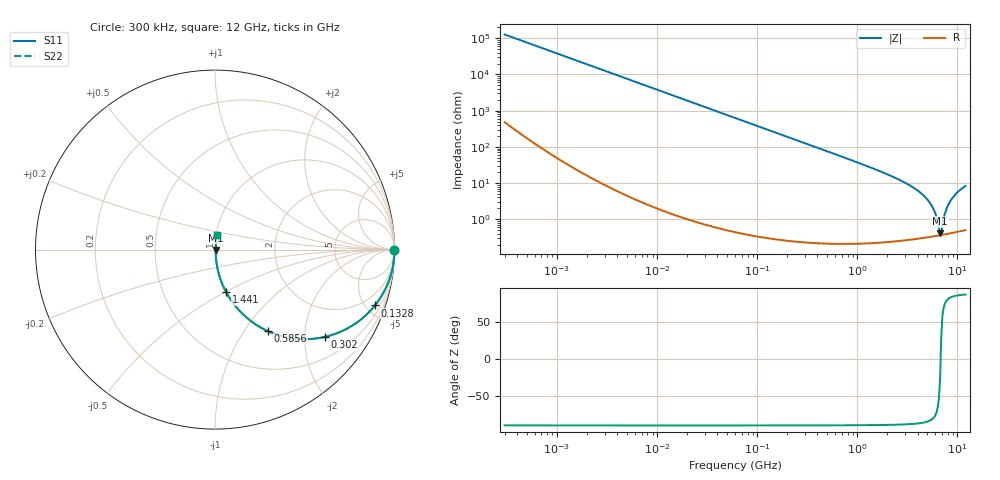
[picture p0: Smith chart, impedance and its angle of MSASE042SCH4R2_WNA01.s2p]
! MSASE042SCH4R2_WNA01  S-PARAMETER MODEL  ( General Type )
! Model Generated by TAIYO YUDEN Corporation (http://www.ty-top.com)
! Version 1.0
! TAIYO YUDEN Control No. 120810
! Copyright(c) 2012 TAIYO YUDEN CO.,LTD. All Rights Reserved.
! Product Description (link to TY-COMPAS)
! https://ds.yuden.co.jp/TYCOMPAS/or/detail?pn=MSASE042SCH4R2BWNA01&u=M
! Products Name : Multilayer Ceramic Capacitors
! Characteristics :
!  Capacitance : 4.2 pF , Rated Voltage : 16V , TCC : CH / C0H
!  Case Size : 0.4 x 0.2 / 0.016 x 0.008 [mm/inch] , Thickness : 0.2 / 0.008 [mm/inch]
!  (Conditions: Temperature = 25 degC , DC Bias Current/Voltage = 0A / 0V)
! External Node Assignments :
!  1  o---| |---o  2
! GND o---------o GND
! Frequency Range : 0.3MHz  -  12000MHz  [ 401 STEP ]
# MHz S RI R 50
! Freq[MHz].  S11 Real  S11 Imag  S21 Real  S21 Imag  S12 Real  S12 Imag  S22 Real  S22 Imag
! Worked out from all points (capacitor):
!   401 points, 300 kHz to 12 GHz, reference 50 ohm
!   read as one part in series: C = 4.19 pF near 316.3 kHz
!   lowest |Z| = 413 mohm at 6.7 GHz (marker M1)
!   series resonance near 6.792 GHz, so ESL is about 130 pH
!   S11 on the Smith chart (normalised r, x): 300 kHz: open; 132.8 MHz: 1.01, -5.72; 302 MHz: 1.00, -2.51; 585.6 MHz: 1.00, -1.29; 1.441 GHz: 1.00, -0.50; 12 GHz: 1.01, +0.17
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0.3  1 -0.000789  3.61e-06 0.000789  3.61e-06 0.000789  1 -0.000789
1.769972  1 -0.00466  2.59e-05 0.00466  2.59e-05 0.00466  1 -0.00466
10.44266  0.9992 -0.0275  0.000769 0.0275  0.000769 0.0275  0.9992 -0.0275
60  0.9756 -0.154  0.0244 0.154  0.0244 0.154  0.9756 -0.154
132.8329  0.8908 -0.3114  0.1092 0.3114  0.1092 0.3114  0.8908 -0.3114
301.9711  0.6118 -0.4864  0.3882 0.4864  0.3882 0.4864  0.6118 -0.4864
353.9943  0.534 -0.4978  0.466 0.4978  0.466 0.4978  0.534 -0.4978
585.5907  0.2938 -0.4539  0.7062 0.4539  0.7062 0.4539  0.2938 -0.4539
894.6982  0.1496 -0.3542  0.8504 0.3542  0.8504 0.3542  0.1496 -0.3542
1441.349  0.0615 -0.2359  0.9385 0.2359  0.9385 0.2359  0.0615 -0.2359
2088.533  0.0286 -0.1598  0.9714 0.1598  0.9714 0.1598  0.0286 -0.1598
3454.93  0.00932 -0.0807  0.9907 0.0807  0.9907 0.0807  0.00932 -0.0807
4747.894  0.00477 -0.0409  0.9952 0.0409  0.9952 0.0409  0.00477 -0.0409
5715.274  0.00374 -0.0196  0.9963 0.0196  0.9963 0.0196  0.00374 -0.0196
6026.253  0.00362 -0.0137  0.9964 0.0137  0.9964 0.0137  0.00362 -0.0137
6524.734  0.00359 -0.00484  0.9964 0.00484  0.9964 0.00484  0.00359 -0.00484
6699.894  0.00362 -0.00197  0.9964 0.00197  0.9964 0.00197  0.00362 -0.00197
7064.448  0.00375 0.00576  0.9963 -0.00576  0.9963 -0.00576  0.00375 0.00576
7648.807  0.00413 0.0162  0.9959 -0.0162  0.9959 -0.0162  0.00413 0.0162
8503.825  0.00507 0.0313  0.9949 -0.0313  0.9949 -0.0313  0.00507 0.0313
9968.853  0.00747 0.0546  0.9925 -0.0546  0.9925 -0.0546  0.00747 0.0546
12000  0.0118 0.0818  0.9882 -0.0818  0.9882 -0.0818  0.0118 0.0818
